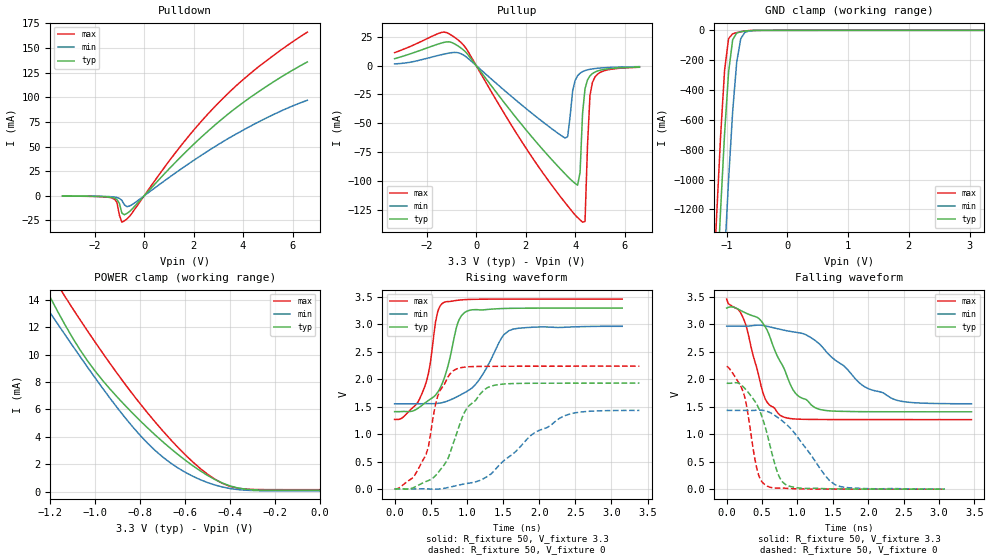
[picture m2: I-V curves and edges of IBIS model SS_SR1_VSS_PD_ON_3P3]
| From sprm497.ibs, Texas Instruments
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|   Model Cell SS_SR1_VSS_PD_ON_3P3
|SR0_VSS_SR1_VSS_PD_ON_3P3
[Model]   SS_SR1_VSS_PD_ON_3P3
Model_type   I/O
Polarity   Non-Inverting
Enable   Active-Low
Vinl =  0.8V
Vinh =  2V
Cref =  5.0000pF
Rref =  100.0000M
Vref =  0V
Vmeas =  1.65
C_comp   2.113745p   2.040636p   2.247812p
[Model Spec]
Vinl   0.8V   0.8V   0.8V
Vinh   2V   2V   2V
[Temperature Range]   25   125   -40
[Voltage Range]   3.3   2.97   3.465
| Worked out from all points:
|   slope of the pulldown table from 0 to 0.495 V, typ, clamps not added: 36.4 ohm
|   slope of the pullup table from 0 to 0.495 V, typ, clamps not added: 34.9 ohm
|   GND clamp passes 1 mA (typ) near -0.57 V on its own axis
|   POWER clamp passes 1 mA (typ) near -0.48 V on its own axis
|   rising waveform, R_fixture 50, V_fixture 3.3: 20-80 % time 244ps typ, 386ps min, 197ps max; typ from 1.41 V to 3.3 V
|   rising waveform, R_fixture 50, V_fixture 0: 20-80 % time 398ps typ, 796ps min, 267ps max; typ from 0 V to 1.93 V
|   falling waveform, R_fixture 50, V_fixture 3.3: 20-80 % time 388ps typ, 716ps min, 265ps max; typ from 3.3 V to 1.41 V
|   falling waveform, R_fixture 50, V_fixture 0: 20-80 % time 271ps typ, 498ps min, 187ps max; typ from 1.93 V to 0 V
[POWER_clamp]
|   voltage   I(typ)   I(min)   I(max)
-3.3V     86.18mA    64.56mA    104.4mA
-1.267V   16.33mA    14.66mA    18.08mA
-1.233V   15.23mA    13.85mA    17mA
-1.2V     14.16mA    13.03mA    16mA
-1.133V   12.14mA    11.42mA    14.2mA
-1V       8.786mA    8.291mA    10.9mA
-866.7mV  6.286mA    5.394mA    7.837mA
-766.7mV  4.65mA     3.535mA    5.745mA
-633.3mV  2.737mA    1.75mA     3.262mA
-500mV    1.189mA    665.2uA    1.278mA
-366.7mV  275.7uA    153.6uA    253.8uA
-11.55fV  94.2uA     52.09uA    142.8uA
[Pulldown]
|   voltage   I(typ)   I(min)   I(max)
-3.3V     -240.7uA   -171.6uA   -267.5uA
-1.3V     -1.697mA   -968uA     -2.239mA
-1.1V     -3.762mA   -1.687mA   -6.637mA
-1V       -7.728mA   -2.567mA   -19.64mA
-900mV    -17.44mA   -4.637mA   -26.73mA
-800mV    -19.19mA   -8.992mA   -25.39mA
-700mV    -17.88mA   -11mA      -23.57mA
-500mV    -13.74mA   -9.146mA   -17.83mA
1.4V      37.42mA    25.57mA    48.03mA
2.9V      72.6mA     50.52mA    91.53mA
4.6V      105.1mA    74.64mA    130.4mA
6.6V      135.8mA    96.92mA    166.1mA
[Pullup]
|   voltage   I(typ)   I(min)   I(max)
-3.3V     6.015mA    1.488mA    11.26mA
-1.4V     19.63mA    9.503mA    28.79mA
-700mV    16.55mA    11.01mA    21.71mA
3.6V      -93.97mA   -62.76mA   -119mA
4.1V      -103.6mA   -8.736mA   -131.8mA
4.2V      -92.66mA   -6.551mA   -133.7mA
4.3V      -41.56mA   -5.211mA   -135.8mA
4.4V      -19.91mA   -4.314mA   -135.1mA
4.5V      -12.4mA    -3.675mA   -69.73mA
4.6V      -8.869mA   -3.197mA   -25.87mA
4.7V      -6.864mA   -2.828mA   -14.55mA
6.6V      -1.25mA    -873.6uA   -1.41mA
[GND_clamp]
|   voltage   I(typ)   I(min)   I(max)
-3.3V     -22.46A    -23.25A    -22.02A
-1.233V   -2.372A    -3.255A    -1.856A
-1.167V   -1.78A     -2.658A    -1.268A
-1.1V     -1.214A    -2.077A    -719.3mA
-1.033V   -694.9mA   -1.519A    -269mA
-966.7mV  -277.7mA   -998.2mA   -54.82mA
-900mV    -62.93mA   -543.8mA   -23.21mA
-833.3mV  -17.83mA   -212.7mA   -15.14mA
-766.7mV  -9.317mA   -55.45mA   -9.115mA
-700mV    -5.152mA   -13.93mA   -4.514mA
-633.3mV  -2.404mA   -4.879mA   -1.658mA
3.233V    94.16uA    65.13uA    142.7uA
[Ramp]
| variable   typ   min   max
dV/dt_f   1.529924/0.7199493n   1.147946/1.235254n   1.775827/0.4961274n
dV/dt_r   1.546938/0.6661015n   1.150875/1.140294n   1.794156/0.4666181n
R_load = 50
[Rising Waveform]
R_fixture = 50
V_fixture = 3.3
V_fixture_min = 2.97
V_fixture_max = 3.465
|   time   V(typ)   V(min)   V(max)
0s        1.409V     1.553V     1.267V
119ps     1.412V     1.553V     1.31V
371ps     1.517V     1.554V     1.716V
469ps     1.615V     1.555V     2.11V
595ps     1.76V      1.56V      3.222V
672ps     1.966V     1.578V     3.394V
882ps     3.053V     1.694V     3.442V
1.022ns   3.252V     1.796V     3.455V
1.582ns   3.293V     2.886V     3.461V
3.15ns    3.298V     2.966V     3.462V
[Rising Waveform]
R_fixture = 50
V_fixture = 0
V_fixture_min = 0
V_fixture_max = 0
|   time   V(typ)   V(min)   V(max)
0s        5.609uV    6.87uV     4.835uV
245ps     14.51mV    -57.33uV   197.3mV
434ps     135.4mV    1.751mV    624.1mV
595ps     286.9mV    -3.079mV   1.687V
833ps     911.9mV    53.47mV    2.172V
994ps     1.458V     97.71mV    2.224V
1.344ns   1.878V     283.7mV    2.236V
1.89ns    1.927V     980.8mV    2.238V
2.366ns   1.928V     1.341V     2.239V
3.388ns   1.929V     1.431V     2.239V
[Falling Waveform]
R_fixture = 50
V_fixture = 3.3
V_fixture_min = 2.97
V_fixture_max = 3.465
|   time   V(typ)   V(min)   V(max)
0s        3.298V     2.969V     3.463V
252ps     3.219V     2.967V     3.059V
455ps     3.109V     2.988V     2.055V
546ps     2.954V     2.974V     1.639V
777ps     2.282V     2.905V     1.329V
973ps     1.745V     2.858V     1.278V
1.309ns   1.454V     2.647V     1.269V
1.932ns   1.411V     1.878V     1.267V
2.366ns   1.41V      1.635V     1.267V
3.458ns   1.409V     1.556V     1.267V
[Falling Waveform]
R_fixture = 50
V_fixture = 0
V_fixture_min = 0
V_fixture_max = 0
|   time   V(typ)   V(min)   V(max)
0s        1.93V      1.434V     2.239V
238ps     1.859V     1.434V     1.752V
294ps     1.778V     1.434V     1.423V
434ps     1.524V     1.439V     332mV
483ps     1.375V     1.439V     163.4mV
560ps     1.061V     1.422V     64.55mV
735ps     248.1mV    1.293V     19.41mV
889ps     53.21mV    1.125V     11.53mV
1.526ns   5.278mV    84.47mV    1.502mV
3.08ns    458.9uV    3.032mV    149.1uV
